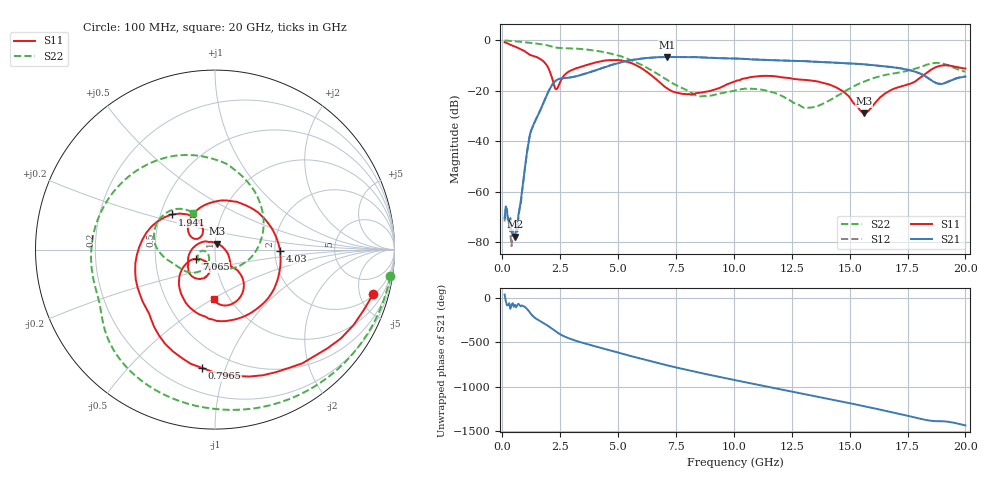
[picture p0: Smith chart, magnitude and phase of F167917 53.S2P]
!  2-Port S-parameters saved by WinCal
! VAR MeasName=S-Parameters (CALIBRATED_DATA) read from VNA (N5242A)
! VAR MeasDate=2016-11-22 9:02:33
! VAR NAME=F167917 53
! VAR FILENAME=F167917 53.S2P
! VAR DATE=2016-11-22 9:02:33
! VAR PHYS_PORTS=1,2
# Hz S DB R 50
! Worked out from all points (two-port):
!   401 points, 100 MHz to 20 GHz, reference 50 ohm
!   highest |S21| = -6.65 dB at 7.115 GHz (marker M1); lowest = -77.9 dB at 547.8 MHz (marker M2)
!   |S21| within 3 dB of the highest: 4.78 GHz to 15.74 GHz (10.96 GHz wide, 107 % of centre)
!   lowest |S11| = -28.9 dB at 15.62 GHz (marker M3), VSWR 1.07, Z = 51.3 + j3.4 ohm
!   |S11| at or under -10 dB: 1.925 GHz to 3.573 GHz (1.648 GHz wide, 60 % of centre); 5.799 GHz to 19.02 GHz (13.23 GHz wide, 107 % of centre); 19.26 GHz to end of sweep
!   |S22| runs from -26.8 to -0.1 dB; largest |S21 - S12| = 0.0038
!   S11 on the Smith chart (normalised r, x): 100 MHz: 2.16, -6.63; 796.5 MHz: 0.35, -0.83; 1.941 GHz: 0.58, +0.25; 4.03 GHz: 2.14, -0.04; 7.065 GHz: 0.81, -0.08; 20 GHz: 0.85, -0.51
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1e8  -0.76 -15.6  -70.45 37.9  -71.82 59.3  -0.10 -8.7
5.4775e8  -2.51 -69.2  -77.86 -79.1  -73.85 -78.7  -0.40 -44.6
7.965e8  -3.57 -96.2  -63.76 -94.7  -65.41 -96.2  -0.62 -63.3
1.1945e9  -5.82 -135.8  -37.39 -165.5  -37.35 -165.1  -1.05 -90.8
1.94075e9  -10.21 140.6  -21.37 50.4  -21.35 50.5  -2.02 -136.0
2.33875e9  -19.45 140.1  -15.86 -23.4  -15.83 -23.4  -2.93 -153.9
3.43325e9  -10.46 55.4  -13.69 -143.9  -13.68 -143.9  -3.51 161.1
4.03025e9  -8.81 -1.4  -11.91 172.2  -11.90 172.3  -4.15 134.8
4.7765e9  -7.84 -60.3  -9.65 119.2  -9.62 119.3  -5.50 99.9
5.42325e9  -8.61 -103.7  -8.09 73.1  -8.04 73.1  -7.40 66.9
6.7665e9  -16.43 -156.4  -6.73 -18.1  -6.72 -18.2  -13.70 -11.6
7.065e9  -18.74 -153.7  -6.67 -37.2  -6.68 -37.3  -15.40 -29.9
7.11475e9  -19.07 -153.0  -6.65 -40.4  -6.66 -40.4  -15.67 -33.1
8.30875e9  -21.31 -119.0  -6.70 -111.7  -6.67 -111.6  -21.50 -95.9
1.005e10  -16.34 -107.2  -7.28 152.5  -7.27 152.6  -19.96 -126.0
1.149275e10  -14.16 -133.3  -7.87 76.9  -7.82 76.8  -20.21 -163.9
1.338325e10  -16.05 -161.3  -8.46 -21.8  -8.44 -21.8  -26.63 -143.6
1.45275e10  -19.24 167.7  -9.00 -81.9  -8.96 -82.0  -21.72 -115.8
1.5622e10  -28.92 67.7  -9.55 -141.6  -9.61 -141.7  -16.42 -125.5
1.67165e10  -20.09 -34.0  -10.52 156.9  -10.56 157.3  -13.45 -148.2
1.885575e10  -10.28 -64.8  -17.31 48.6  -17.18 49.2  -9.00 153.4
2e10  -11.21 -90.7  -14.44 1.0  -14.32 1.0  -12.49 121.7
